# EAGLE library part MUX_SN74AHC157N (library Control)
QUAD 2 LINE TO 1 LINE DATA SELECTORS/MULTIPLEXERS
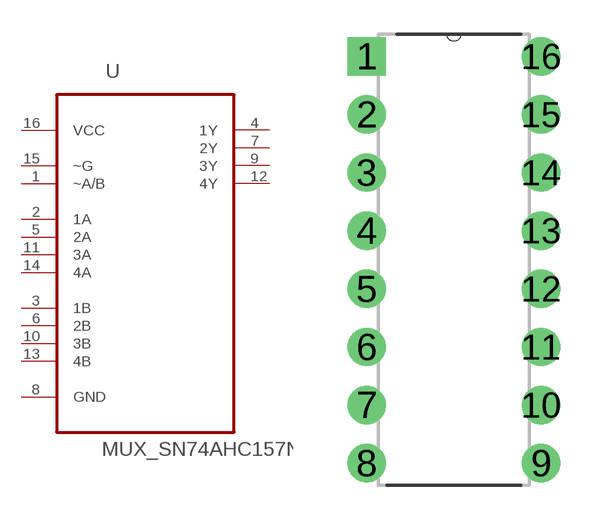
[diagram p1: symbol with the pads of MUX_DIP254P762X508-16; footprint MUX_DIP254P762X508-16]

Designator prefix U

## MUX_SN74AHC157N (MPN: SN74AHC157N; OC_FARNELL: 1741531; OC_NEWARK: 34R8444; PACKAGE: 16-DIP; SUPPLIER: Texas Instruments)  [MUX_DIP254P762X508-16]
1  ~A/B  in
2  1A  in
3  1B  in
4  1Y  out
5  2A  in
6  2B  in
7  2Y  out
8  GND  pas
9  3Y  out
10  3B  in
11  3A  in
12  4Y  out
13  4B  in
14  4A  in
15  ~G  in
16  VCC  pwr

## Footprint MUX_DIP254P762X508-16 (pad centres in mm)
drill 1.118 square: 1 -7.62,17.78
drill 1.118: 2 -7.62,15.24; 3 -7.62,12.7; 4 -7.62,10.16; 5 -7.62,7.62; 6 -7.62,5.08; 7 -7.62,2.54; 8 -7.62,0; 9 0,0; 10 0,2.54; 11 0,5.08; 12 0,7.62; 13 0,10.16; 14 0,12.7; 15 0,15.24; 16 0,17.78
